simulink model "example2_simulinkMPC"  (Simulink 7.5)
settings: Solver=ode45  SolverMode=SingleTasking  StartTime=0.0  StopTime=10000  FixedStep=100  RelTol=1e-3
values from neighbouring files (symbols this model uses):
  A = [0 0.0001 0;0 0 0.0001;-2.4 -0.25 -0.005]    [example_3_7_1_podklad.m]    (also in example_3_7_2_podklad.m; example_3_7_3_podklad.m)
  B = [0;0;3]    [example_3_7_1_podklad.m]    (also in example_3_7_2_podklad.m; example_3_7_3_podklad.m)
  C = [1 0 0]    [example_3_7_1_podklad.m]    (also in example_3_7_2_podklad.m; example_3_7_3_podklad.m)
  D = 0    [example_3_7_1_podklad.m]    (also in example_3_7_2_podklad.m; example_3_7_3_podklad.m)
  Ts = 100    [example_3_7_1_podklad.m]    (also in example_3_7_2_podklad.m; example_3_7_3_podklad.m)
undefined symbols (not defined in the file or in its folder): sigbuilder_block
libraries: mpclib x1, simulink x1

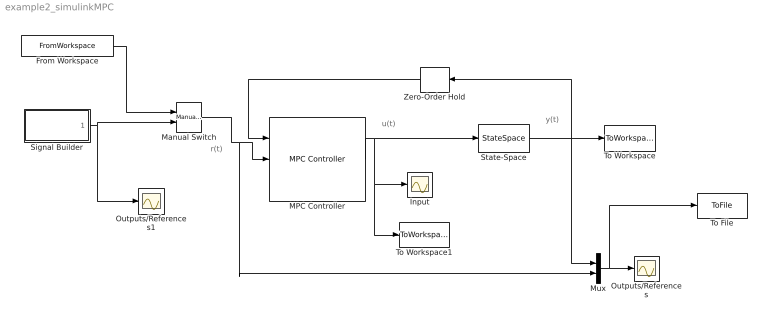
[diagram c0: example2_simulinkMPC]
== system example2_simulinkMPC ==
  note: u(t)
  note: y(t)
  note: r(t)
  From Workspace : FromWorkspace  VariableName=[(Ts*(0:length(r)-1))' r']  SampleTime=Ts  Interpolate=off  OutputAfterFinalValue=Setting to zero
  Input : Scope
  MPC Controller : mpclib/MPC Controller  SystemSampleTime=-1  mpcobj=mpc_controller  n_mv=0  x0=[]  ref_from_ws=off  ref_signal_name=[]  ref_preview=on  md_from_ws=off  md_signal_name=[]  md_preview=on  from_project=off  md_inport=on  mv_inport=off  lims_inport=off  switch_inport=off  enable_value=0  project_file=MPCtask.mat  task_name=MPC Controller  is_multiple=0
  Manual Switch : simulink/Signal Routing/Manual Switch  SystemSampleTime=-1  sw=0  action=0  varsize=off
  Mux : Mux  Inputs=2
  Outputs/References : Scope
  Outputs/References1 : Scope
  Signal Builder : Subsystem  Tag=STV Subsys  LoadFcn=sigbuilder_block('load');  StartFcn=sigbuilder_block('start');  StopFcn=sigbuilder_block('stop');  ClipboardFcn=sigbuilder_block('clipboard');
  State-Space : StateSpace  A=A  B=B  C=C  D=D
  To File : ToFile  Filename=simoutMPC  MatrixName=simoutMPC
  To Workspace : ToWorkspace  VariableName=y  SampleTime=-1  SaveFormat=Array
  To Workspace1 : ToWorkspace  VariableName=u  SampleTime=-1  SaveFormat=Array
  Zero-Order Hold : ZeroOrderHold  SampleTime=Ts
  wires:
  MPC Controller/1 -> Input/1, To Workspace1/1, State-Space/1
  State-Space/1 -> To Workspace/1, Mux/1, Zero-Order Hold/1
  Mux/1 -> Outputs/References/1, To File/1
  Zero-Order Hold/1 -> MPC Controller/1
  Manual Switch/1 -> MPC Controller/2, Mux/2
  From Workspace/1 -> Manual Switch/1
  Signal Builder/1(Signal 2) -> Manual Switch/2, Outputs/References1/1

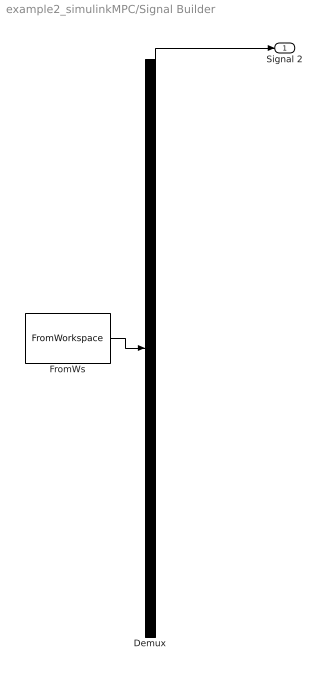
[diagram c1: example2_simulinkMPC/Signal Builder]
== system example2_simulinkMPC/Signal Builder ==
  Demux : Demux  Tag=STV Demux  Outputs=1
  FromWs : FromWorkspace  Tag=STV FromWs  VariableName=tuvar  SampleTime=0  SigBuilderData=DataTag0  VnvData=DataTag1
  Signal 2 : Outport  Tag=STV Outport
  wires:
  FromWs/1 -> Demux/1
  Demux/1 -> Signal 2/1
